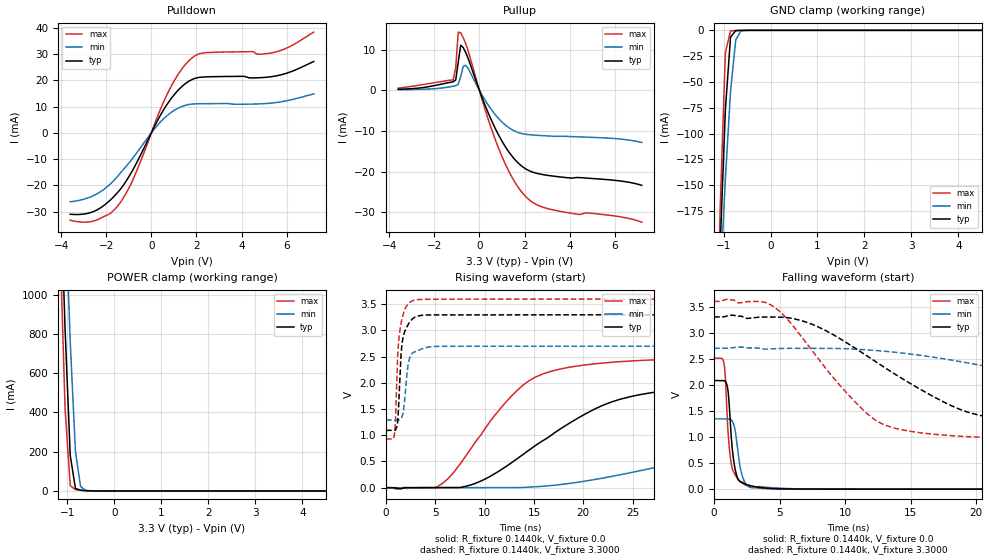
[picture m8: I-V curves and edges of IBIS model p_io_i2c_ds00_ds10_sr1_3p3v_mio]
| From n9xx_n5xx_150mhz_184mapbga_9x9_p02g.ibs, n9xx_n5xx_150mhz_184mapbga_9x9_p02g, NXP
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[Model] p_io_i2c_ds00_ds10_sr1_3p3v_mio
|   Model p_io_i2c_ds00_ds10_sr1_3p3v_mio
| This model was characterised for following simulation conditions:
| External (pad) voltage:
|   - Typ: 3.3V,   - Min: 2.7V,   - Max: 3.6V
| Library cells for typ/min/max conditions are connected as defined below:
|  pad - External Pad
|  ipp_do_lv - Core Input
|  ipp_obe_lv - Output Buffer Enable
|  IOGC - NC
|  REFH3V3 - REFH3V3
|  REFL3V3 - REFL3V3
|  ZI - NC
|  abut_ncal_vddio[1] - vddio
|  abut_ncal_vddio[2] - vddio
|  abut_ncal_vddio[3] - vssio
|  abut_ncal_vddio[4] - vddio
|  abut_ncal_vddio[5] - vddio
|  abut_ncal_vddio[6] - vssio
|  abut_pcal_vddio[1] - vssio
|  abut_pcal_vddio[2] - vssio
|  abut_pcal_vddio[3] - vddio
|  abut_pcal_vddio[4] - vssio
|  abut_pcal_vddio[5] - vssio
|  abut_pcal_vddio[6] - vddio
|  ipp_do_1p8v - ipp_do_1p8v
|  ipp_dse_lv[0] - 0
|  ipp_dse_lv[1] - 0
|  ipp_eftd_lv - NC
|  ipp_ina_mux_vddio - NC
|  ipp_ina_mux_vddio[0] - NC
|  ipp_ina_mux_vddio[1] - NC
|  ipp_ina_r0_vddio - NC
|  ipp_ina_r0a_vddio - NC
|  ipp_ina_r0b_vddio - NC
|  ipp_ina_r0c_vddio - NC
|  ipp_ina_r0d_vddio - NC
|  ipp_ina_r0e_vddio - NC
|  ipp_ina_r0f_vddio - NC
|  ipp_ina_r300_vddio - NC
|  ipp_ina_r300a_vddio - NC
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Model_type I/O
Polarity   Non-Inverting
Enable   Active-High
Vinl =   0.9900V
Vinh =   2.3100V
Vmeas =  1.6500V
Cref =   30.0000pF
Rref =   1.0000M
Vref =   3.3000V
C_comp   1.4149pF   1.3702pF   1.4746pF
|C_comp_pullup   0.5857pF   0.6311pF   0.5571pF
|C_comp_pulldown   0.7313pF   0.7412pF   0.7168pF
[Model Spec]
| variable   typ   min   max
Vinh   2.3100V   1.8900V   2.5200V
Vinl   0.9900V   0.8100V   1.0800V
[Temperature Range]   25.0000   0.1250k   -40.0000
[Voltage Range]   3.3000V   2.7000V   3.6000V
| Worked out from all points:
|   slope of the pulldown table from 0 to 0.495 V, typ, clamps not added: 61.3 ohm
|   slope of the pullup table from 0 to 0.495 V, typ, clamps not added: 71.7 ohm
|   GND clamp passes 1 mA (typ) near -0.75 V on its own axis
|   POWER clamp passes 1 mA (typ) near -0.57 V on its own axis
|   rising waveform, R_fixture 0.1440k, V_fixture 0.0: 20-80 % time 11.1ns typ, 24ns min, 6.55ns max; typ from 0 V to 2.08 V
|   rising waveform, R_fixture 0.1440k, V_fixture 3.3000: 20-80 % time 446ps typ, 479ps min, 464ps max; typ from 1.09 V to 3.3 V
|   falling waveform, R_fixture 0.1440k, V_fixture 0.0: 20-80 % time 437ps typ, 497ps min, 411ps max; typ from 2.08 V to 0 V
|   falling waveform, R_fixture 0.1440k, V_fixture 3.3000: 20-80 % time 8.94ns typ, 19.6ns min, 5.38ns max; typ from 3.3 V to 1.09 V
[Pulldown]
|Voltage   I(typ)   I(min)   I(max)
-3.6V     -30.97mA   -26.22mA   -33.25mA
-2.5V     -29.69mA   -23.6mA    -33.39mA
-1.84V    -25.73mA   -19.61mA   -30.76mA
-1.4V     -21.71mA   -15.56mA   -26.77mA
-850mV    -14.57mA   -9.916mA   -18.47mA
140mV     2.472mA    1.548mA    3.283mA
800mV     12.12mA    7.253mA    16.41mA
1.35V     17.58mA    10.01mA    24.26mA
1.79V     20.21mA    10.91mA    28.4mA
2.45V     21.27mA    11.08mA    30.48mA
5.42V     21.48mA    11.4mA     30.56mA
7.2V      27.13mA    14.79mA    38.3mA
[Pullup]
|Voltage   I(typ)   I(min)   I(max)
-3.6V     265.1uA    141.9uA    552.1uA
-1.16V    2.117mA    1.022mA    2.595mA
-1.05V    2.581mA    1.145mA    5.627mA
-940mV    6.922mA    1.451mA    14.34mA
-830mV    11.11mA    3.398mA    14.14mA
-720mV    10.54mA    5.878mA    12.98mA
-610mV    9.33mA     6.194mA    11.53mA
820mV     -10.67mA   -6.749mA   -13.83mA
1.48V     -16.43mA   -9.783mA   -21.74mA
2.03V     -19.25mA   -10.79mA   -26.01mA
3.24V     -21.09mA   -11.29mA   -29.39mA
7.2V      -23.38mA   -12.83mA   -32.45mA
[GND_clamp]
|Voltage   I(typ)   I(min)   I(max)
-3.6V     -4.327A    -3.181A    -5.901A
-1.18V    -358.9mA   -350.6mA   -379.3mA
-1.07V    -208.2mA   -244.2mA   -170.8mA
-960mV    -76.59mA   -144.3mA   -21.58mA
-850mV    -6.561mA   -58.74mA   -508.1uA
-740mV    -273.3uA   -9.382mA   -183.5uA
-630mV    -73.8uA    -593.1uA   -76.7uA
-410mV    -3.432uA   -9.016uA   -2.096uA
7.2V      0A         0A         0A
[POWER_clamp]
|Voltage   I(typ)   I(min)   I(max)
-3.6V     20.44A     18.76A     22.48A
-1.16V    1.647A     2.216A     1.289A
-1.05V    823.6mA    1.482A     419.2mA
-940mV    180.4mA    758.9mA    26.72mA
-830mV    12.56mA    202.9mA    6.794mA
-720mV    3.422mA    22.23mA    3.58mA
-610mV    1.373mA    2.923mA    1.344mA
7.2V      0A         0A         0A
[Ramp]
| variable   typ   min   max
dV/dt_r  1.2491/11.0986n   0.8048/23.9975n   1.5059/6.5476n
dV/dt_f  1.3242/8.9358n   0.8439/19.6377n   1.6016/5.3768n
R_load = 0.1440k
[Rising Waveform]
R_fixture= 0.1440k
V_fixture= 0.0
V_fixture_min= 0.0
V_fixture_max= 0.0
|time   V(typ)   V(min)   V(max)
0s        3.241nV    240.6nV    11.14nV
5.186ns   -105.3uV   -197.1uV   19.56mV
9.066ns   82.28mV    -39.46uV   873.6mV
12.04ns   388.5mV    247.9uV    1.61V
14.5ns    716.4mV    9.399mV    2.04V
21.75ns   1.552V     174.2mV    2.375V
31.82ns   1.915V     568mV      2.468V
43.38ns   2.016V     972.3mV    2.497V
54.84ns   2.053V     1.156V     2.506V
133.4ns   2.082V     1.341V     2.51V
[Rising Waveform]
R_fixture= 0.1440k
V_fixture= 3.3000
V_fixture_min= 2.7000
V_fixture_max= 3.6000
|time   V(typ)   V(min)   V(max)
0s        1.093V     1.29V      930.6mV
865.4ps   1.093V     1.29V      1.031V
944.1ps   1.1V       1.29V      1.244V
1.212ns   1.344V     1.29V      2.633V
1.444ns   2.312V     1.3V       3.06V
1.585ns   2.685V     1.339V     3.197V
1.79ns    2.921V     1.501V     3.341V
2.328ns   3.141V     2.431V     3.526V
3.204ns   3.275V     2.615V     3.589V
133.4ns   3.3V       2.7V       3.6V
[Falling Waveform]
R_fixture= 0.1440k
V_fixture= 0.0
V_fixture_min= 0.0
V_fixture_max= 0.0
|time   V(typ)   V(min)   V(max)
0s        2.082V     1.348V     2.51V
767.5ps   2.08V      1.348V     2.395V
862.1ps   2.064V     1.347V     2.127V
1.064ns   1.882V     1.348V     1.092V
1.234ns   1.295V     1.34V      619.2mV
1.42ns    693.9mV    1.288V     365.1mV
1.768ns   227.2mV    821mV      209.7mV
2.283ns   109.5mV    162.6mV    94.21mV
3.599ns   29.3mV     43.49mV    15.54mV
133.4ns   159.9nV    3.244uV    33.63nV
[Falling Waveform]
R_fixture= 0.1440k
V_fixture= 3.3000
V_fixture_min= 2.7000
V_fixture_max= 3.6000
|time   V(typ)   V(min)   V(max)
0s        3.3V       2.7V       3.6V
4.346ns   3.299V     2.688V     3.528V
7.487ns   3.159V     2.7V       2.649V
12.08ns   2.483V     2.662V     1.363V
17.59ns   1.663V     2.496V     1.035V
20.73ns   1.391V     2.356V     991.2mV
25.39ns   1.253V     2.127V     960.8mV
35.46ns   1.151V     1.671V     939.3mV
45.73ns   1.118V     1.473V     933.5mV
133.4ns   1.093V     1.294V     930.6mV
